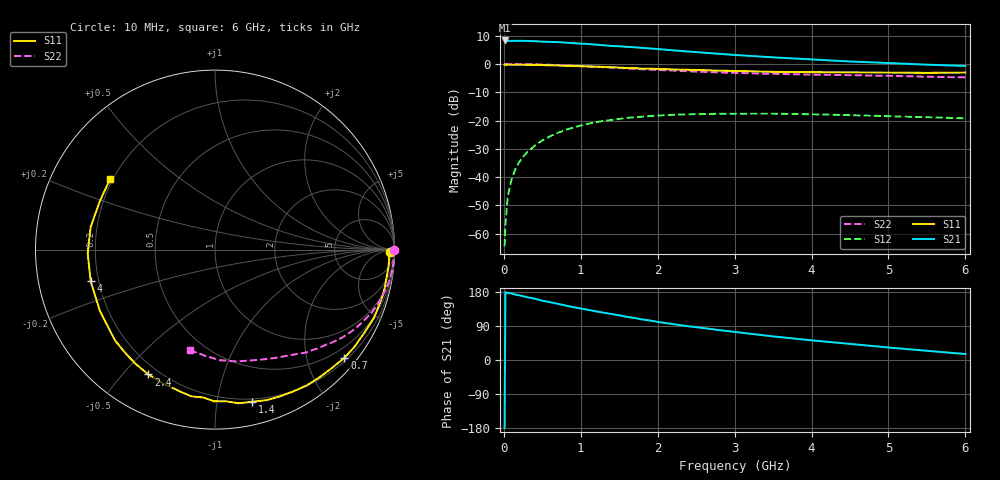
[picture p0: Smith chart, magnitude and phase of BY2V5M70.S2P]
! SIEMENS Small Signal Semiconductors
! BFY420
! Si NPN RF SIEGET Grounded Emitter Transistor in MICRO-X
! VCE = 2.5 V  IC = 0.7 mA
! Common Emitter S-Parameters:  October  1996
# GHz  S  MA  R  50
!  f  S11  S21  S12  S22
! GHz  MAG  ANG  MAG  ANG  MAG  ANG  MAG  ANG
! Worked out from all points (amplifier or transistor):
!   36 points, 10 MHz to 6 GHz, reference 50 ohm
!   highest |S21| = 8.3 dB at 10 MHz (marker M1)
!   |S21| within 3 dB of that: start of sweep to 1.981 GHz
!   unconditionally stable (mu >= 1): 4.702 GHz to end of sweep
!   at 250 MHz: K = 0.03, MSG = 20.5 dB, |S12| = -32.8 dB
!   at 1.4 GHz: K = 0.18, MSG = 13.1 dB, |S12| = -19.8 dB
!   at 6 GHz: K = 1.38, MAG = 5.6 dB, |S12| = -19.2 dB
!   S11 on the Smith chart (normalised r, x): 10 MHz: 60, -26; 700 MHz: 0.26, -2.73; 1.4 GHz: 0.18, -1.26; 2.4 GHz: 0.16, -0.59; 4 GHz: 0.17, -0.12; 6 GHz: 0.19, +0.29
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0.01  0.9723 -0.7  2.602 -179.3  0.0006 103.1  0.9992 -0.2
0.02  0.963 -1.2  2.597 178.9  0.0014 92.6  0.9936 -0.5
0.05  0.9725 -3.0  2.569 177.1  0.0045 86.3  0.9988 -1.4
0.1  0.971 -6.0  2.556 175.8  0.009 88.0  0.9945 -2.8
0.15  0.9686 -8.7  2.56 172.4  0.0138 82.7  0.9967 -4.2
0.25  0.9692 -14.4  2.559 168.3  0.0228 80.8  0.9932 -6.9
0.4  0.9643 -23.2  2.531 162.0  0.0357 75.3  0.9842 -11.0
0.5  0.9523 -29.1  2.479 156.4  0.0445 72.4  0.9751 -13.6
0.7  0.94 -39.9  2.432 148.3  0.0603 65.7  0.9555 -18.8
0.9  0.9192 -50.9  2.332 139.5  0.075 58.5  0.9294 -23.7
1.1  0.9017 -61.6  2.253 132.1  0.0878 52.4  0.9029 -28.3
1.4  0.8726 -76.2  2.077 121.2  0.1023 43.6  0.8622 -34.6
1.6  0.8474 -85.9  2.007 113.8  0.1113 38.2  0.832 -38.5
1.8  0.8264 -94.6  1.921 107.0  0.1167 33.2  0.8059 -41.9
2.2  0.8006 -111.0  1.742 94.7  0.1263 24.4  0.7646 -48.6
2.4  0.7886 -118.1  1.657 89.0  0.1286 20.9  0.7409 -51.6
2.8  0.762 -131.3  1.51 78.9  0.1316 14.1  0.7071 -57.2
3.5  0.7263 -152.1  1.308 62.3  0.132 5.0  0.6687 -66.1
4  0.7148 -165.7  1.203 51.9  0.1289 -0.1  0.6477 -72.7
4.5  0.7096 -178.3  1.105 42.5  0.1244 -4.0  0.6335 -79.5
5.5  0.6959 157.5  0.971 24.3  0.1143 -7.8  0.5947 -95.1
6  0.7047 146.1  0.921 15.8  0.1092 -7.3  0.5782 -103.8
